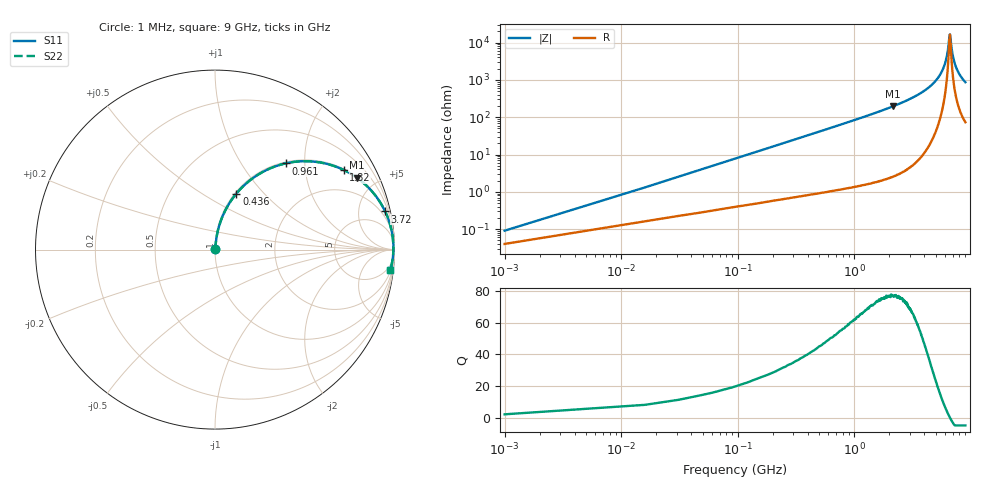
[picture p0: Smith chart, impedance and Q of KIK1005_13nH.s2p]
!version-3
!date-01.2023
!Series
# MHz S RI R 50
!Freq ReS11 ImS11 ReS21 ImS21 ReS12 ImS12 ReS22 ImS22
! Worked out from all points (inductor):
!   601 points, 1 MHz to 9 GHz, reference 50 ohm
!   read as one part in series: L = 13 nH near 46 MHz
!   highest Q = 77.1 at 2.15 GHz (marker M1), where L = 14.5 nH
!   self-resonance near 6.62 GHz
!   S11 on the Smith chart (normalised r, x): 1 MHz: 1.00, +0.00; 436 MHz: 1.02, +0.72; 961 MHz: 1.03, +1.60; 1.82 GHz: 1.04, +3.21; 3.72 GHz: 1.17, +8.88; 9 GHz: 2, -17
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1  0.000407 0.000816  0.9996 -0.000816  0.9996 -0.000816  0.000407 0.000816
61  0.00562 0.0494  0.9944 -0.0494  0.9944 -0.0494  0.00562 0.0494
106  0.0115 0.0853  0.9885 -0.0853  0.9885 -0.0853  0.0115 0.0853
226  0.0385 0.1766  0.9615 -0.1766  0.9615 -0.1766  0.0385 0.1766
436  0.1193 0.3124  0.8807 -0.3124  0.8807 -0.3124  0.1193 0.3124
661  0.2337 0.4135  0.7663 -0.4135  0.7663 -0.4135  0.2337 0.4135
961  0.3931 0.4803  0.6069 -0.4803  0.6069 -0.4803  0.3931 0.4803
1520  0.629 0.4762  0.371 -0.4762  0.371 -0.4762  0.629 0.4762
1820  0.7175 0.4436  0.2825 -0.4436  0.2825 -0.4436  0.7175 0.4436
2150  0.7902 0.4007  0.2098 -0.4007  0.2098 -0.4007  0.7902 0.4007
3020  0.9028 0.2891  0.0973 -0.2891  0.0973 -0.2891  0.9028 0.2891
3720  0.9481 0.2126  0.0519 -0.2126  0.0519 -0.2126  0.9481 0.2126
4520  0.9754 0.1409  0.0246 -0.1409  0.0246 -0.1409  0.9754 0.1409
5420  0.9897 0.0738  0.0103 -0.0738  0.0103 -0.0738  0.9897 0.0738
6020  0.9934 0.0353  0.00658 -0.0353  0.00658 -0.0353  0.9934 0.0353
6290  0.994 0.0192  0.00598 -0.0192  0.00598 -0.0192  0.994 0.0192
6570  0.994 0.00301  0.00595 -0.00301  0.00595 -0.00301  0.994 0.00301
6630  0.994 -0.000302  0.00601 0.000302  0.00601 0.000302  0.994 -0.000302
7020  0.993 -0.0211  0.00696 0.0211  0.00696 0.0211  0.993 -0.0211
7520  0.9907 -0.0459  0.00933 0.0459  0.00933 0.0459  0.9907 -0.0459
8130  0.9862 -0.0745  0.0138 0.0745  0.0138 0.0745  0.9862 -0.0745
9000  0.9777 -0.1112  0.0223 0.1112  0.0223 0.1112  0.9777 -0.1112
